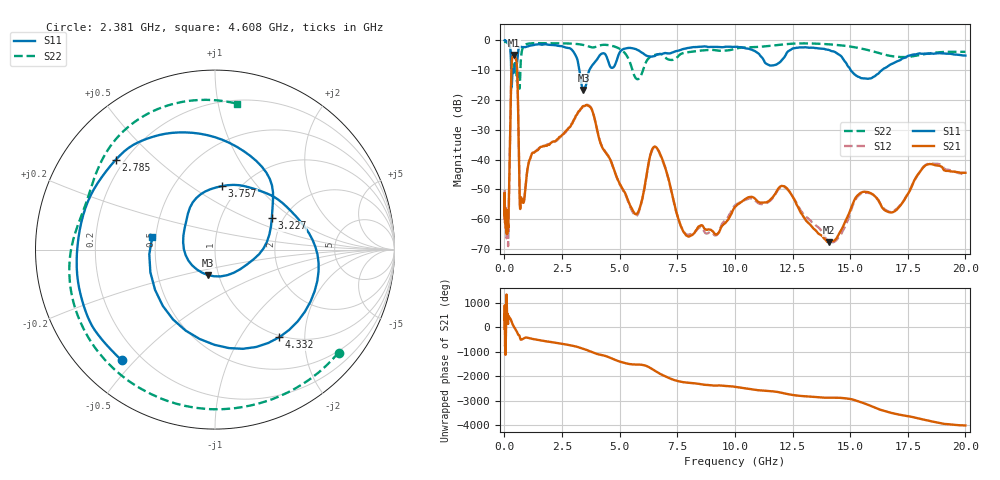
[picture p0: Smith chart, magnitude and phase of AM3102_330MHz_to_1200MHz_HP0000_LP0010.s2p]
! Date/Time: Tue, Sep 11, 2018 5:08 PM
! Network Analyzer: Agilent Technologies E8362B Rev: A.07.50.63
! Sweep from 0.010 to 20.000 GHz, 1601 Points, Sweep Type: LOG
! Power Supply: 4.950 V, 0.000 A
# Hz S DB R 50
!freq MagS11 AngS11 MagS21 AngS21 MagS12 AngS12 MagS22 AngS22
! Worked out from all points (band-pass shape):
!   1601 points, 10 MHz to 20 GHz, reference 50 ohm
!   highest |S21| = -4.84 dB at 402.8 MHz (marker M1); lowest = -67.8 dB at 14.07 GHz (marker M2)
!   |S21| within 3 dB of the highest: 316.5 MHz to 535.3 MHz (218.8 MHz wide, 51.4 % of centre)
!   lowest |S11| = -16.6 dB at 3.432 GHz (marker M3), VSWR 1.35, Z = 44.5 - j12.9 ohm
!   |S11| at or under -10 dB: 294.9 MHz to 355.8 MHz (60.91 MHz wide, 18.7 % of centre); 3.256 GHz to 3.684 GHz (427.6 MHz wide, 12.3 % of centre); 15.03 GHz to 16.38 GHz (1.349 GHz wide, 8.59 % of centre)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
!   |S22| runs from -16.2 to -0.2 dB; largest |S21 - S12| = 0.0084
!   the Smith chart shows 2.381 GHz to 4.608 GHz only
!   S11 on the Smith chart (normalised r, x): 2.381 GHz: 0.13, -0.46; 2.785 GHz: 0.17, +0.37; 3.227 GHz: 1.75, +0.70; 3.757 GHz: 0.83, +0.67; 4.332 GHz: 0.97, -1.50; 4.608 GHz: 0.48, +0.08
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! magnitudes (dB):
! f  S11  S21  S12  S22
! 10 MHz  0.0  -51.4  -51.5  -0.2
! 35.55 MHz  0.0  -60.9  -61.5  -0.4
! 126.4 MHz  -0.4  -64.5  -61.5  -0.8
! 164.9 MHz  -0.8  -62.7  -66.7  -1.1
! 402.8 MHz  -10.8  -4.8  -4.9  -8.9
! 447.2 MHz  -9.0  -5.2  -5.3  -7.6
! 559.1 MHz  -6.8  -11.2  -11.3  -13.5
! 682.6 MHz  -2.2  -56.5  -56.3  -13.0
! 1.59 GHz  -1.4  -35.7  -35.7  -0.9
! 2.381 GHz  -1.9  -32.5  -32.8  -1.0
! 2.785 GHz  -2.5  -29.4  -29.4  -1.0
! 3.227 GHz  -8.8  -23.8  -24.0  -1.3
! 3.432 GHz  -16.6  -22.0  -22.2  -1.5
! 3.757 GHz  -9.0  -22.6  -22.6  -2.3
! 4.332 GHz  -4.4  -36.9  -36.8  -1.5
! 4.608 GHz  -9.0  -40.2  -40.3  -1.7
! 5.652 GHz  -2.8  -58.1  -58.7  -12.1
! 6.58 GHz  -4.9  -35.8  -36.0  -4.8
! 7.92 GHz  -2.6  -65.6  -65.2  -4.0
! 12.09 GHz  -6.2  -48.9  -49.1  -1.4
! 14.07 GHz  -3.2  -67.8  -67.4  -1.3
! 20 GHz  -5.1  -44.4  -45.1  -3.8
